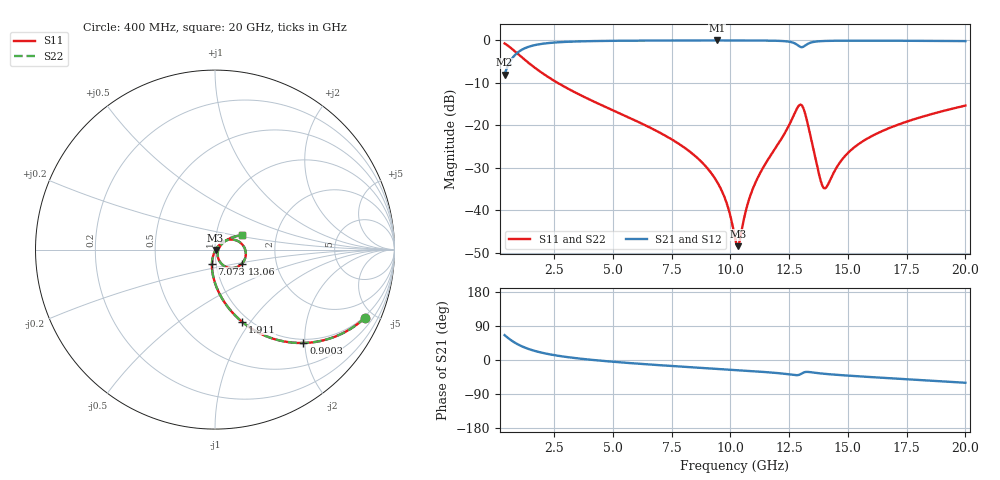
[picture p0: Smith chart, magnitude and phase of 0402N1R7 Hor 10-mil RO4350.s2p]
# GHz S MA R 50
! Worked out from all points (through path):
!   1960 points, 400 MHz to 20 GHz, reference 50 ohm
!   highest |S21| = -0.03 dB at 9.435 GHz (marker M1); lowest = -8.1 dB at 400 MHz (marker M2)
!   group delay of S21, straight-line fit = 12.4 ps
!   lowest |S11| = -48.5 dB at 10.32 GHz (marker M3), VSWR 1.01, Z = 50.3 - j0.179 ohm
!   |S11| at or under -10 dB: 2.652 GHz to end of sweep
!   |S22| runs from -48.5 to -0.7 dB; largest |S21 - S12| = 0
!   S11 on the Smith chart (normalised r, x): 400 MHz: 0.92, -4.46; 900.3 MHz: 0.92, -1.97; 1.911 GHz: 0.92, -0.91; 7.073 GHz: 0.96, -0.15; 13.06 GHz: 1.33, -0.22; 20 GHz: 1.33, +0.22
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0.4  0.9185 -24.3  0.3952 65.6  0.3952 65.6  0.9185 -24.3
0.9002552  0.7165 -46.6  0.6969 43.4  0.6969 43.4  0.7165 -46.6
1.910771  0.4285 -69.5  0.9023 20.3  0.9023 20.3  0.4285 -69.5
3.671669  0.2233 -86.4  0.9729 3.2  0.9729 3.2  0.2233 -86.4
6.943338  0.08354 -101.8  0.9938 -13.5  0.9938 -13.5  0.08354 -101.8
7.073405  0.07991 -102.2  0.994 -14.0  0.994 -14.0  0.07991 -102.2
8.51414  0.0433 -106.1  0.9958 -19.8  0.9958 -19.8  0.0433 -106.1
9.434609  0.02166 -105.0  0.9962 -23.5  0.9962 -23.5  0.02166 -105.0
9.864829  0.01169 -98.1  0.9961 -25.1  0.9961 -25.1  0.01169 -98.1
10.205  0.004647 -64.2  0.9959 -26.5  0.9959 -26.5  0.004647 -64.2
10.31506  0.003777 -28.1  0.9958 -26.9  0.9958 -26.9  0.003777 -28.1
10.75528  0.01229 40.8  0.9952 -28.7  0.9952 -28.7  0.01229 40.8
11.11547  0.02254 46.9  0.9943 -30.2  0.9943 -30.2  0.02254 46.9
12.63624  0.1199 27.1  0.945 -39.0  0.945 -39.0  0.1199 27.1
12.89638  0.1676 0.5  0.8654 -39.6  0.8654 -39.6  0.1676 0.5
13.05646  0.1692 -27.9  0.8313 -35.0  0.8313 -35.0  0.1692 -27.9
13.46667  0.06395 -69.3  0.9474 -32.6  0.9474 -32.6  0.06395 -69.3
13.83686  0.02267 -48.2  0.9773 -35.4  0.9773 -35.4  0.02267 -48.2
14.02695  0.01813 -13.3  0.9827 -36.6  0.9827 -36.6  0.01813 -13.3
15.07749  0.04941 39.4  0.9904 -41.5  0.9904 -41.5  0.04941 39.4
16.73834  0.09217 38.4  0.9893 -48.0  0.9893 -48.0  0.09217 38.4
20  0.1705 28.1  0.979 -60.1  0.979 -60.1  0.1705 28.1
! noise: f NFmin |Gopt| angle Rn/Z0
0.4  0.001286  0.8028  4.532  0.001352
2.571  0.005075  0.6801  8.306  0.003053
4.752  0.008077  0.6384  13.52  0.004159
6.933  0.01084  0.6152  18.83  0.005105
9.104  0.01379  0.6085  24.05  0.006257
11.29  0.02037  0.6644  29.23  0.01092
13.47  0.06752  0.8666  34.8  0.09912
15.64  0.02599  0.6504  39.7  0.01257
17.82  0.02529  0.6087  44.35  0.01036
20  0.02676  0.5969  48.88  0.01025
